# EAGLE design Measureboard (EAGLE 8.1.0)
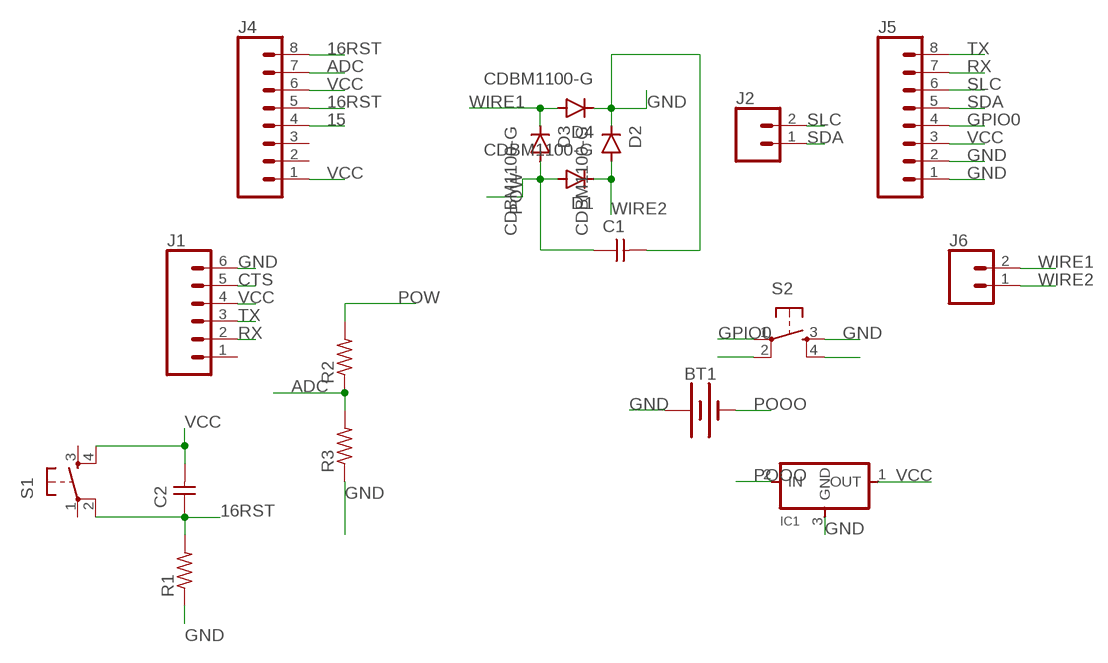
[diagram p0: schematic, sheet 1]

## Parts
BT1  BATTERY-20MM_SMD  [BATTCON_20MM]
C1  CAP-UNPOLARIZED  [C1206]
C2  CAP-UNPOLARIZEDFAB  [C1206FAB]
D1  CDBM1100-G  [MINI-SMA]
D2  CDBM1100-G  [MINI-SMA]
D3  CDBM1100-G  [MINI-SMA]
D4  CDBM1100-G  [MINI-SMA]
IC1  REGULATORSOT23  [SOT23]
J1  CONN_06LONGPADS  [1X06_LONGPADS]
J2  CONN_02PTH3  [1X02_LONGPADS]
J4  CONN_08LONGPADS  [1X08_LONGPADS]
J5  CONN_08LONGPADS  [1X08_LONGPADS]
J6  CONN_02PTH3  [1X02_LONGPADS]
R1  RES-US1206FAB  [R1206FAB]
R2  RES-US1206FAB  [R1206FAB]
R3  RES-US1206FAB  [R1206FAB]
S1  6MM_SWITCH6MM_SWITCH  [6MM_SWITCH]
S2  6MM_SWITCH6MM_SWITCH  [6MM_SWITCH]

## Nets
15: J4.4
16RST: C2.1 J4.5 J4.8 R1.2 S1.2(P1)
ADC: J4.7 R2.1 R3.2
CTS: J1.5
GND: BT1.1(+) C1.2 D2.KATHODE D4.KATHODE IC1.3(GND) J1.6 J5.1 J5.2 R1.1 R3.1 S2.3(S)
GPIO0: J5.4 S2.1(P)
N$2: S2.4(S1)
N$3: S2.2(P1)
POOO: BT1.2(-) IC1.2(IN)
POW: C1.1 D1.ANODE D3.ANODE R2.2
RX: J1.2 J5.7
SDA: J2.1 J5.5
SLC: J2.2 J5.6
TX: J1.3 J5.8
VCC: C2.2 IC1.1(OUT) J1.4 J4.1 J4.6 J5.3 S1.4(S1)
WIRE1: D3.KATHODE D4.ANODE J6.2
WIRE2: D1.KATHODE D2.ANODE J6.1
Unconnected: J1.1 J4.2 J4.3 S1.1(P) S1.3(S)

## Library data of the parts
BT1 = SparkFun-Batteries:BATTERY: Battery - Single Cell; PROD_ID: BATT-11519
C1 C2 = fab:CAP-UNPOLARIZED
D1-D4 = fab:CDBM1100-G: Diode schottky 100V 1A mini-SMA as found in the fablab inventory
IC1 = fab:REGULATOR
J1 = SparkFun-Connectors:CONN_06: Multi connection point. Often used as Generic Header-pin footprint for 0.1 inch spaced/style header connections On any of the 0.1 inch spaced packages, you can populate with these: Break Away Headers - Straight (PRT-00116) Break Away Male Headers - Right Angle (PRT-00553) Female Headers (PRT-00115)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
J2 J6 = SparkFun-Connectors:CONN_02: Multi connection point. Often used as Generic Header-pin footprint for 0.1 inch spaced/style header connections
J4 J5 = SparkFun-Connectors:CONN_08: Multi connection point. Often used as Generic Header-pin footprint for 0.1 inch spaced/style header connections On any of the 0.1 inch spaced packages, you can populate with these: Break Away Headers - Straight (PRT-00116) Break Away Male Headers - Right Angle (PRT-00553) Female Headers (PRT-00115)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
R1-R3 = fab:RES-US: Resistor (US Symbol)
S1 S2 = fab:6MM_SWITCH: OMRON SWITCH

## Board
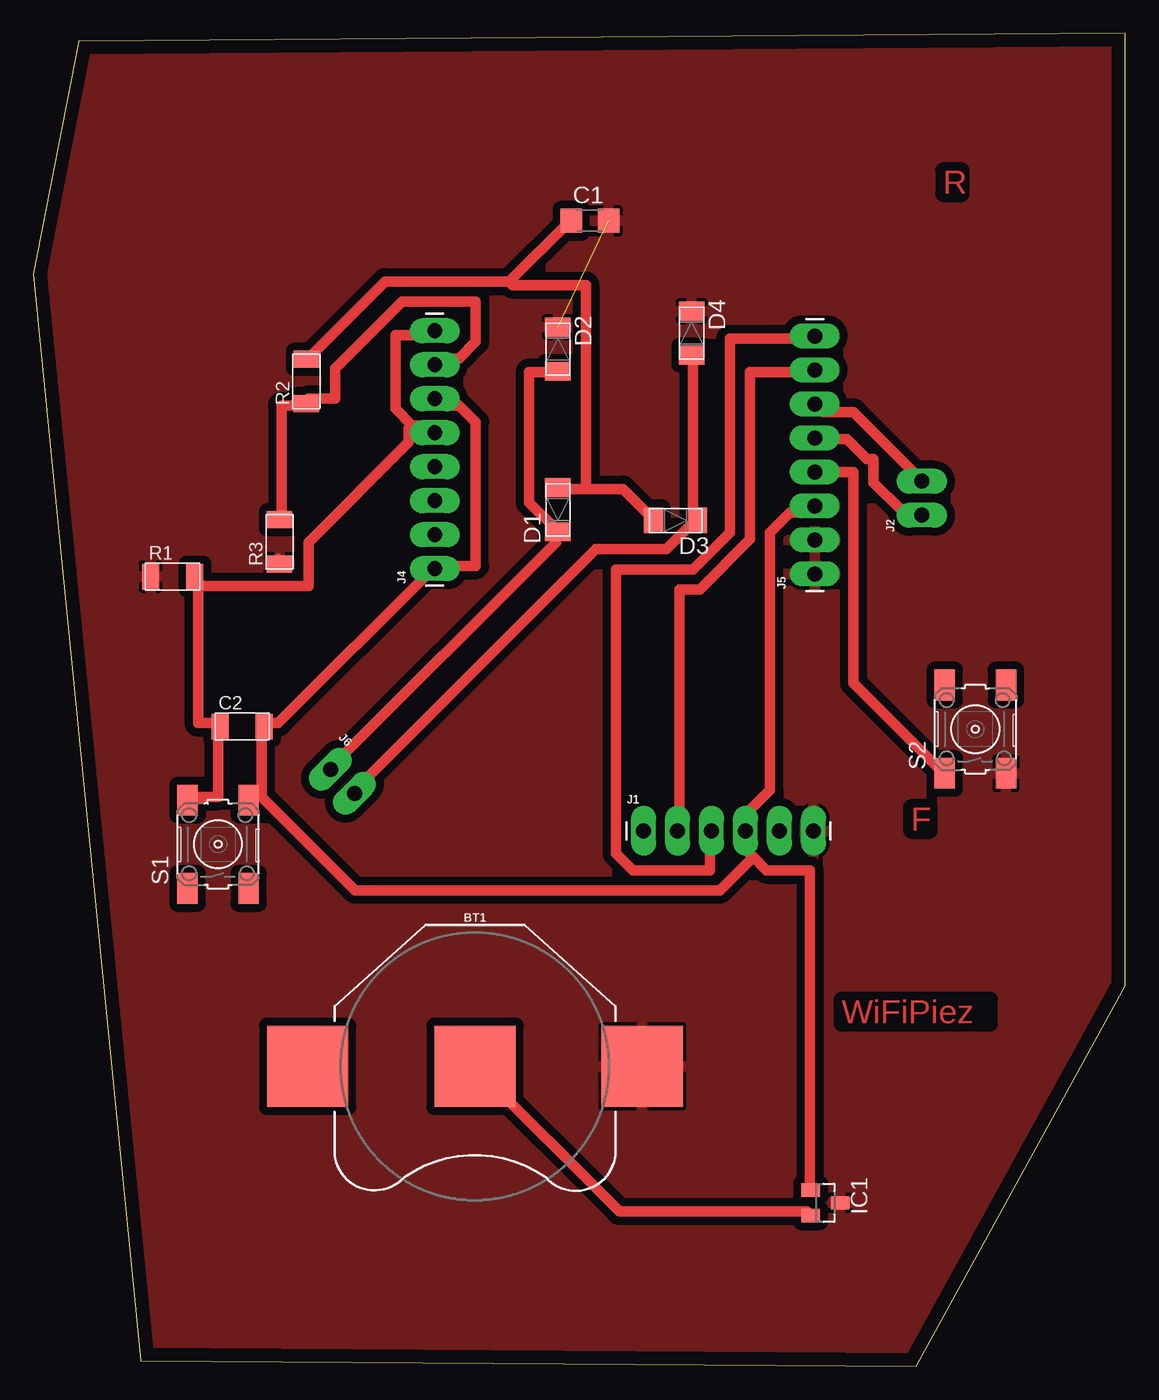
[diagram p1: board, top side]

Size 81.6 x 99.6 mm. Coordinates in mm from the lower left corner, seen from the top.
Outline: 0,81.6 8,0.4 66,0 81.6,28.4 81.6,99.6 3.4,99 0,81.6
Copper layers (1*16): Top 0.035mm / dielectric 1.5mm / Bottom 0.035mm
Design rules "default *": minimum track width 0.8mm, minimum drill 24mil, track to track 0.6mm, track to pad 0.6mm, pad to pad 0.6mm, via to via 0.4mm, smd to smd 0.4mm, copper to edge 40mil, drill to drill 8mil, minimum pad ring 10mil, minimum via ring 8mil, stop-mask expansion 4mil, vias tented up to drill 0mil, thermal gap 10mil

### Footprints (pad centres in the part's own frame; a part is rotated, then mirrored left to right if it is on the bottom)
BATTCON_20MM = smd 6.07 x 6.07: 1 -12.5,0; 2 0,0; 3 12.5,0
C1206 = smd 1.6 x 1.8: 1 -1.4,0; 2 1.4,0
C1206FAB = smd 1.27 x 1.905: 1 -1.651,0; 2 1.651,0
MINI-SMA = smd 1.4 x 1.9: ANODE 1.65,0; KATHODE -1.65,0
SOT23 = smd 1 x 1.4: 1 -0.95,-1.1; 2 0.95,-1.1; 3 0,1.1
1X06_LONGPADS = drill 1.118 pad 1.88 long: 1 0,0; 2 2.54,0; 3 5.08,0; 4 7.62,0; 5 10.16,0; 6 12.7,0
1X02_LONGPADS = drill 1.118 pad 1.88 long: 1 0,0; 2 2.54,0
1X08_LONGPADS = drill 1.118 pad 1.88 long: 1 0,0; 2 2.54,0; 3 5.08,0; 4 7.62,0; 5 10.16,0; 6 12.7,0; 7 15.24,0; 8 17.78,0
R1206FAB = smd 1.27 x 1.905: 1 -1.651,0; 2 1.651,0
6MM_SWITCH = smd 2.286 x 1.524: 1 -3.302,2.286; 2 3.302,2.286; 3 -3.302,-2.286; 4 3.302,-2.286

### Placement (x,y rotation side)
BT1  33,22.4 180 top
C1  41.6,85.6 0 top
C2  15.6,47.8 0 top
D1  39.2,64 90 top
D2  39.2,76 270 top
D3  48,63.2 180 top
D4  49.2,77.2 270 top
IC1  59.2,12.2 270 top
J1  45.6,40 0 top
J2  66.4,63.6 90 top
J4  30,59.6 90 top
J5  58.4,59.2 90 top
J6  22.2,44.6 315 top
R1  10.4,59 0 top
R2  20.4,73.6 90 top
R3  18.4,61.6 90 top
S1  13.8,39 90 top
S2  70.4,47.6 90 top

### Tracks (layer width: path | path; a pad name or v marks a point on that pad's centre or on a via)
16RST
  Top 0.8: 30.05,77.3 J4.8 29.8,77.05 27.05,77.05 27.05,71.55 28.3,70.3 | 28.3,70.3 29.3,70.3 29.8,69.8 J4.5 | S1.2 11.55,42.55 13.8,42.55 13.8,47.8 C2.1 13.55,48.05 12.3,48.05 12.3,58.8 R1.2 12.55,58.3 20.55,58.3 20.55,61.55 28.05,69.05 28.05,70.05 28.3,70.3
ADC
  Top 0.8: R3.2 18.55,63.3 18.55,71.8 20.3,71.8 R2.1 20.55,72.3 22.55,72.3 22.55,74.55 27.55,79.55 33.05,79.55 33.05,76.55 31.8,75.3 30.3,75.3 30.05,75.05 J4.7
GND  (1 unrouted)
  Top 0.8: 18.55,59.8 R3.1 18.3,60.3
  pour Top: 90,100.4 90,-0.8 0.6,-0.8 1,100.8 1,100.4
GPIO0
  Top 0.8: S2.1 68.05,44.3 61.3,51.05 61.3,66.8 58.55,66.8 J5.4
POOO
  Top 0.8: IC1.2 57.8,11.55 43.8,11.55 33.05,22.3 BT1.2
POW
  Top 0.8: 20.55,75.3 R2.2 20.8,75.55 26.3,81.05 35.55,81.05 | 41.3,65.55 39.3,65.55 D1.ANODE | 41.3,65.55 44.05,65.55 46.3,63.3 D3.ANODE | 35.55,81.05 40.05,85.55 C1.1 | 41.3,65.55 41.3,80.8 35.8,80.8 35.55,81.05
RX
  Top 0.8: J1.2 48.3,40.05 48.3,58.05 49.8,58.05 53.55,61.8 53.55,74.3 58.3,74.3 J5.7
SDA
  Top 0.8: J2.1 66.3,63.8 66.05,64.05 64.8,64.05 62.8,66.05 62.8,67.8 62.3,67.8 60.8,69.3 58.55,69.3 J5.5
SLC
  Top 0.8: J5.6 58.55,71.8 59.05,71.3 61.3,71.3 66.3,66.3 J2.2
TX
  Top 0.8: J1.3 50.55,39.8 50.55,37.05 44.8,37.05 43.55,38.3 43.55,59.55 49.3,59.55 52.05,62.3 52.05,76.8 58.3,76.8 J5.8
VCC
  Top 0.8: 17.05,42.55 17.05,47.8 C2.2 17.55,48.05 18.3,48.05 29.8,59.55 J4.1 30.3,59.8 33.05,59.8 33.05,70.55 31.8,71.8 30.55,71.8 30.05,72.3 J4.6 | 17.05,42.55 16.3,42.55 S1.4 | 53.8,38.05 53.3,38.55 53.3,39.8 J1.4 53.3,40.3 53.3,41.3 55.05,43.05 55.05,62.3 56.55,63.8 58.05,63.8 58.3,64.05 J5.3 | 53.8,38.05 54.8,37.05 58.05,37.05 58.05,13.3 IC1.1 | 17.05,42.55 24.05,35.55 51.3,35.55 53.8,38.05
WIRE1
  Top 0.8: D4.ANODE 49.3,75.55 49.3,63.3 49.55,63.3 D3.KATHODE 49.3,63.05 47.3,61.05 42.05,61.05 24.05,43.05 J6.2
WIRE2
  Top 0.8: D2.ANODE 39.05,74.3 37.05,74.3 37.05,64.55 39.05,62.55 D1.KATHODE 39.05,62.05 39.05,61.55 22.3,44.8 J6.1

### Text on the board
Top: R | F | WiFiPiez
